FUNCTION_BLOCK "FB_CABINET_7P7-R22"
TITLE =Control cabinet 7P7-R22
{ S7_language := '9(1) Angielski (Stany Zjednoczone)  11.01.2022  09:45:15' }
VERSION : 0.1


VAR
  SM : STRUCT
   GeneralError : BOOL ;
   GeneralWarning : BOOL ;
   CtrlVoltageON : BOOL ;
   Auto : BOOL ;
   Manual : BOOL ;
   Local : BOOL ;
   Remote : BOOL ;
   CtrlRelease : BOOL ;
   CtrlRelease_A : BOOL ;
   res11 : BOOL ;
   res12 : BOOL ;
   res13 : BOOL ;
   res14 : BOOL ;
   res15 : BOOL ;
   LackCooling : BOOL ;
   LackHeating : BOOL ;
  END_STRUCT ;
  FM : STRUCT
   EnergyCounterFuse : BOOL ;
   ExternalVoltage400VAC : BOOL ;
   ControlVoltage24VDC : BOOL ;
   ControlVoltage230VAC_MS : BOOL ;
   CabinetCoolingFuse : BOOL ;
   ProfiNetSwitchFault : BOOL ;
   MainSwitchFault : BOOL ;
   ExcessTemperature : BOOL ;
   ESTOP : BOOL ;
   FireAlarmPreWarning : BOOL ;
   FireAlarm : BOOL ;
   MainSwitchEmgPower : BOOL ;
   NormElecBefMainSwitch : BOOL ;
   EmgElecBefMainSwitch : BOOL ;
   res16 : BOOL ;
   res17 : BOOL ;
  END_STRUCT ;
  CTRL : STRUCT
   ResetFault : BOOL ;
   ResetESTOP : BOOL ;
   LampTest : BOOL ;
   AutoStart : BOOL ;
   AutoStop : BOOL ;
   res05 : BOOL ;
   res06 : BOOL ;
   res07 : BOOL ;
   res10 : BOOL ;
   res11 : BOOL ;
   res12 : BOOL ;
   res13 : BOOL ;
   res14 : BOOL ;
   res15 : BOOL ;
   res16 : BOOL ;
   res17 : BOOL ;
  END_STRUCT ;
  CTRL_HMI : STRUCT
   ResetFault : BOOL ;
   Auto : BOOL ;
   Manual : BOOL ;
   res03 : BOOL ;
   res04 : BOOL ;
   res05 : BOOL ;
   res06 : BOOL ;
   res07 : BOOL ;
   ProductionOn : BOOL ;
   ProductionBreak : BOOL ;
   PlantOn : BOOL ;
   PlantOff : BOOL ;
   res14 : BOOL ;
   res15 : BOOL ;
   LackCooling : BOOL ;
   LackHeating : BOOL ;
  END_STRUCT ;
  EC : "UDT_EC";	//Energy Counter
END_VAR
VAR_TEMP
  ERROR_REL : BOOL ;
END_VAR
BEGIN
NETWORK
TITLE =STATUS



NETWORK
TITLE =CONTROL VOLTAGE ON
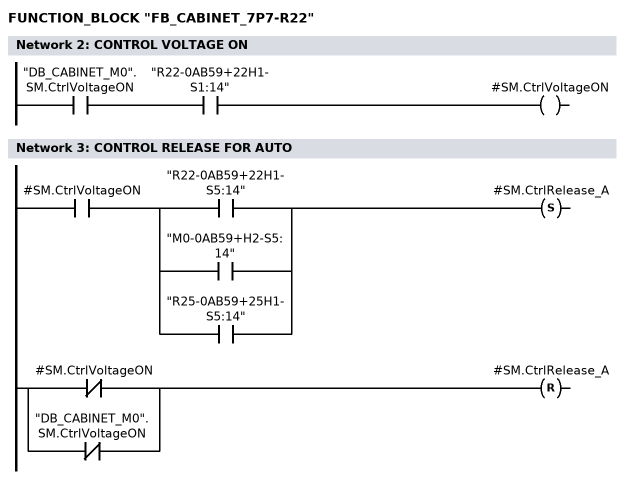
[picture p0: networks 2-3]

      U     "DB_CABINET_M0".SM.CtrlVoltageON;
      U     "R22-0AB59+22H1-S1:14";
      =     #SM.CtrlVoltageON;
NETWORK
TITLE =CONTROL RELEASE FOR AUTO

      U     #SM.CtrlVoltageON;
      U(    ;
      O     "R22-0AB59+22H1-S5:14";
      O     "M0-0AB59+H2-S5:14";
      O     "R25-0AB59+25H1-S5:14";
      )     ;
      S     #SM.CtrlRelease_A;
      U(    ;
      ON    #SM.CtrlVoltageON;
      ON    "DB_CABINET_M0".SM.CtrlVoltageON;
      )     ;
      R     #SM.CtrlRelease_A;
      NOP   0;
NETWORK
TITLE =AUTO/MANUAL MODE

      U(    ;
      U     "R22-0AB59+22H1-S2:14";
      S     #SM.Auto;
      U     "R22-0AB59+22H1-S2:22";
      R     #SM.Auto;
      U     #SM.Auto;
      )     ;
      NOT   ;
      =     #SM.Manual;
NETWORK
TITLE =LOCAL/REMOTE MODE

      U(    ;
      U     "DB_CABINET_M0".SM.Remote;
      S     #SM.Remote;
      U     "DB_CABINET_M0".SM.Local;
      R     #SM.Remote;
      U     #SM.Remote;
      )     ;
      NOT   ;
      =     #SM.Local;
NETWORK
TITLE =CONTROL RELEASE FROM CABINET
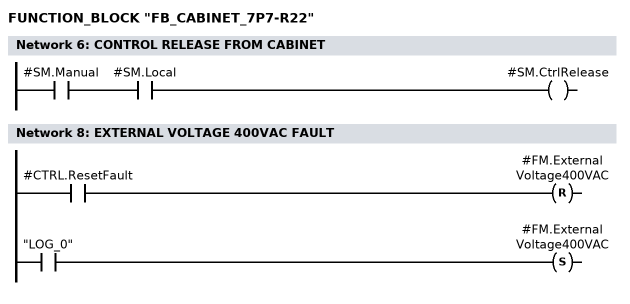
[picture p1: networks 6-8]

      U     #SM.Manual;
      U     #SM.Local;
      =     #SM.CtrlRelease;
NETWORK
TITLE =FAULTS



NETWORK
TITLE =EXTERNAL VOLTAGE 400VAC FAULT

      U     #CTRL.ResetFault;
      R     #FM.ExternalVoltage400VAC;
      U     "LOG_0";
      S     #FM.ExternalVoltage400VAC;
      NOP   0;
NETWORK
TITLE =CONTROL VOLTAGE 24V DC FAULT

      U     #CTRL.ResetFault;
      R     #FM.ControlVoltage24VDC;
      U(    ;
      O(    ;
      UN    "R22-0DC43+22H1-F1:7";
      L     S5T#300MS;
      SE    "T_R22-0DC43+22H1-F1";
      NOP   0;
      NOP   0;
      NOP   0;
      U     "T_R22-0DC43+22H1-F1";
      )     ;
      O(    ;
      UN    "R22-0DC43+22H1-F2:7";
      L     S5T#300MS;
      SE    "T_R22-0DC43+22H1-F2";
      NOP   0;
      NOP   0;
      NOP   0;
      U     "T_R22-0DC43+22H1-F2";
      )     ;
      )     ;
      S     #FM.ControlVoltage24VDC;
      NOP   0;
NETWORK
TITLE =CONTROL VOLTAGE 230VAC BEFORE MAIN SWITCH FAULT
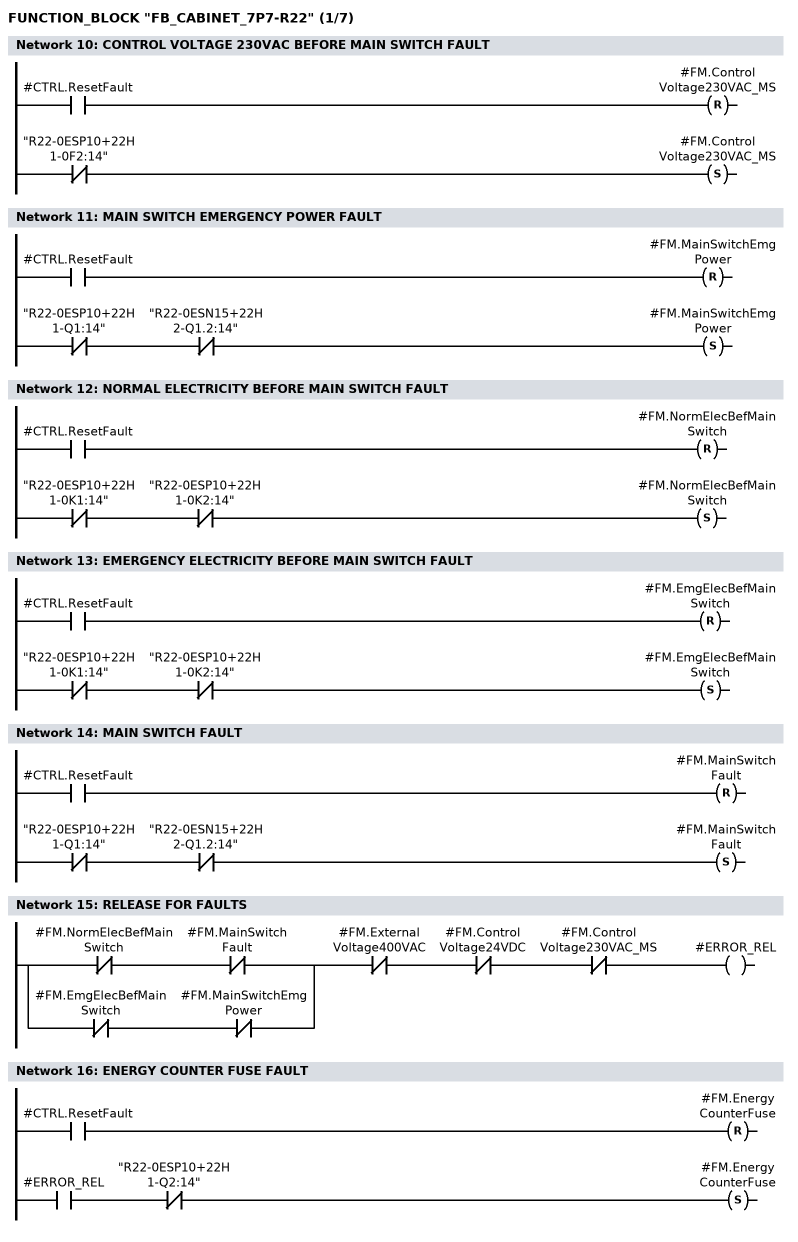
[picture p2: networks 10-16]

      U     #CTRL.ResetFault;
      R     #FM.ControlVoltage230VAC_MS;
      UN    "R22-0ESP10+22H1-0F2:14";
      S     #FM.ControlVoltage230VAC_MS;
      NOP   0;
NETWORK
TITLE =MAIN SWITCH EMERGENCY POWER FAULT

      U     #CTRL.ResetFault;
      R     #FM.MainSwitchEmgPower;
      UN    "R22-0ESP10+22H1-Q1:14";
      UN    "R22-0ESN15+22H2-Q1.2:14";
      S     #FM.MainSwitchEmgPower;
      NOP   0;
NETWORK
TITLE =NORMAL ELECTRICITY BEFORE MAIN SWITCH FAULT

      U     #CTRL.ResetFault;
      R     #FM.NormElecBefMainSwitch;
      UN    "R22-0ESP10+22H1-0K1:14";
      UN    "R22-0ESP10+22H1-0K2:14";
      S     #FM.NormElecBefMainSwitch;
      NOP   0;
NETWORK
TITLE =EMERGENCY ELECTRICITY BEFORE MAIN SWITCH FAULT

      U     #CTRL.ResetFault;
      R     #FM.EmgElecBefMainSwitch;
      UN    "R22-0ESP10+22H1-0K1:14";
      UN    "R22-0ESP10+22H1-0K2:14";
      S     #FM.EmgElecBefMainSwitch;
      NOP   0;
NETWORK
TITLE =MAIN SWITCH FAULT

      U     #CTRL.ResetFault;
      R     #FM.MainSwitchFault;
      UN    "R22-0ESP10+22H1-Q1:14";
      UN    "R22-0ESN15+22H2-Q1.2:14";
      S     #FM.MainSwitchFault;
      NOP   0;
NETWORK
TITLE =RELEASE FOR FAULTS

      U(    ;
      UN    #FM.NormElecBefMainSwitch;
      UN    #FM.MainSwitchFault;
      O     ;
      UN    #FM.EmgElecBefMainSwitch;
      UN    #FM.MainSwitchEmgPower;
      )     ;
      UN    #FM.ExternalVoltage400VAC;
      UN    #FM.ControlVoltage24VDC;
      UN    #FM.ControlVoltage230VAC_MS;
      =     #ERROR_REL;
NETWORK
TITLE =ENERGY COUNTER FUSE FAULT

      U     #CTRL.ResetFault;
      R     #FM.EnergyCounterFuse;
      U     #ERROR_REL;
      UN    "R22-0ESP10+22H1-Q2:14";
      S     #FM.EnergyCounterFuse;
      NOP   0;
NETWORK
TITLE =CABINET COOLING FUSE FAULT
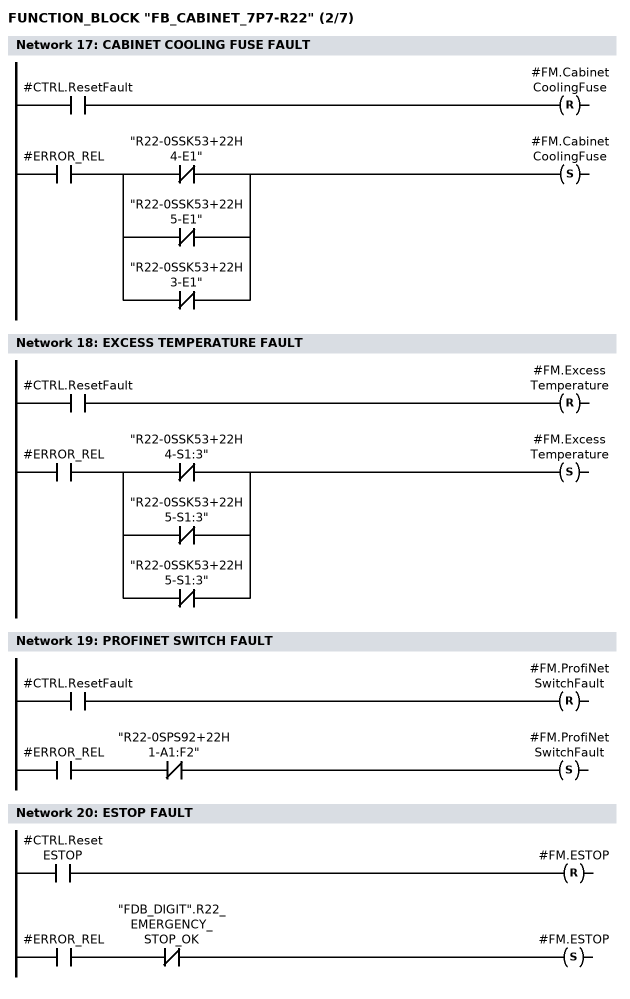
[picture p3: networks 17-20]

      U     #CTRL.ResetFault;
      R     #FM.CabinetCoolingFuse;
      U     #ERROR_REL;
      U(    ;
      ON    "R22-0SSK53+22H4-E1";
      ON    "R22-0SSK53+22H5-E1";
      ON    "R22-0SSK53+22H3-E1";
      )     ;
      S     #FM.CabinetCoolingFuse;
      NOP   0;
NETWORK
TITLE =EXCESS TEMPERATURE FAULT

      U     #CTRL.ResetFault;
      R     #FM.ExcessTemperature;
      U     #ERROR_REL;
      U(    ;
      ON    "R22-0SSK53+22H4-S1:3";
      ON    "R22-0SSK53+22H5-S1:3";
      ON    "R22-0SSK53+22H5-S1:3";
      )     ;
      S     #FM.ExcessTemperature;
      NOP   0;
NETWORK
TITLE =PROFINET SWITCH FAULT

      U     #CTRL.ResetFault;
      R     #FM.ProfiNetSwitchFault;
      U     #ERROR_REL;
      UN    "R22-0SPS92+22H1-A1:F2";
      S     #FM.ProfiNetSwitchFault;
      NOP   0;
NETWORK
TITLE =ESTOP FAULT

      U     #CTRL.ResetESTOP;
      R     #FM.ESTOP;
      U     #ERROR_REL;
      UN    "FDB_DIGIT".R22_EMERGENCY_STOP_OK;
      S     #FM.ESTOP;
      NOP   0;
NETWORK
TITLE =GENERAL FAULT / WARNING
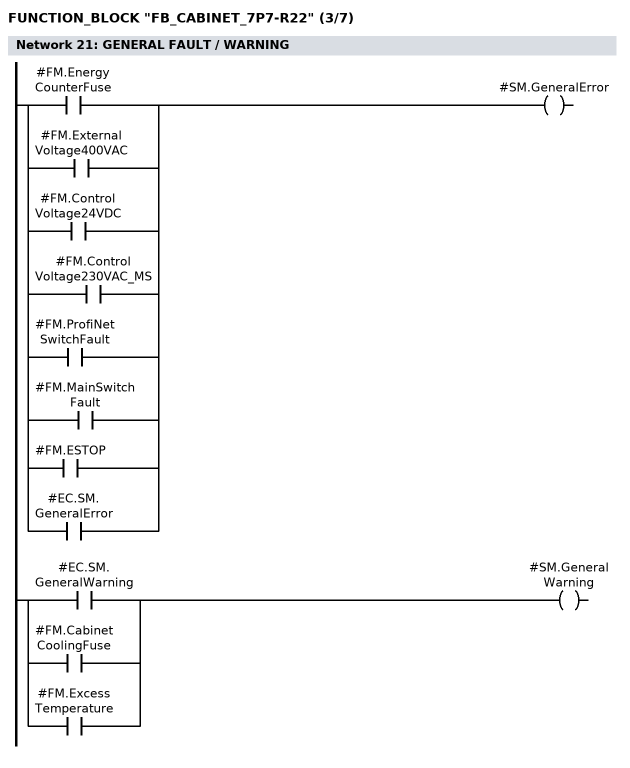
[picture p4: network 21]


      U     #FM.EnergyCounterFuse;
      O     #FM.ExternalVoltage400VAC;
      O     #FM.ControlVoltage24VDC;
      O     #FM.ControlVoltage230VAC_MS;
      O     #FM.ProfiNetSwitchFault;
      O     #FM.MainSwitchFault;
      O     #FM.ESTOP;
      O     #EC.SM.GeneralError;
      =     #SM.GeneralError;


      U     #EC.SM.GeneralWarning;
      O     #FM.CabinetCoolingFuse;
      O     #FM.ExcessTemperature;
      =     #SM.GeneralWarning;

NETWORK
TITLE =CONTROL SIGNALS



NETWORK
TITLE =RESET FAULT
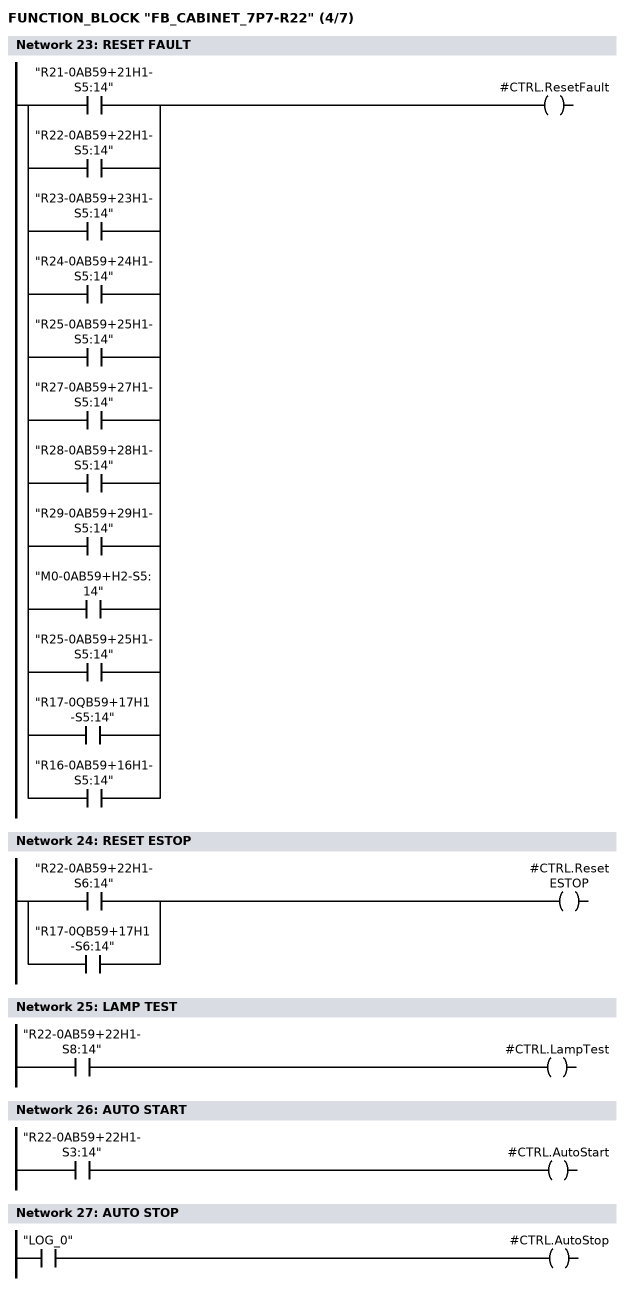
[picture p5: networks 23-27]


      O     "R21-0AB59+21H1-S5:14";
      O     "R22-0AB59+22H1-S5:14";
      O     "R23-0AB59+23H1-S5:14";
      O     "R24-0AB59+24H1-S5:14";
      O     "R25-0AB59+25H1-S5:14";
      O     "R27-0AB59+27H1-S5:14";
      O     "R28-0AB59+28H1-S5:14";
      O     "R29-0AB59+29H1-S5:14";
      O     "M0-0AB59+H2-S5:14";
      O     "R25-0AB59+25H1-S5:14";
      O     "R17-0QB59+17H1-S5:14";
      O     "R16-0AB59+16H1-S5:14";
      =     #CTRL.ResetFault;
NETWORK
TITLE =RESET ESTOP



      O     "R22-0AB59+22H1-S6:14";
      O     "R17-0QB59+17H1-S6:14";
      =     #CTRL.ResetESTOP;
NETWORK
TITLE =LAMP TEST



      U     "R22-0AB59+22H1-S8:14";
      =     #CTRL.LampTest;
NETWORK
TITLE =AUTO START



      U     "R22-0AB59+22H1-S3:14";
      =     #CTRL.AutoStart;
NETWORK
TITLE =AUTO STOP



      U     "LOG_0";
      =     #CTRL.AutoStop;
NETWORK
TITLE =BUTTON LAMPS
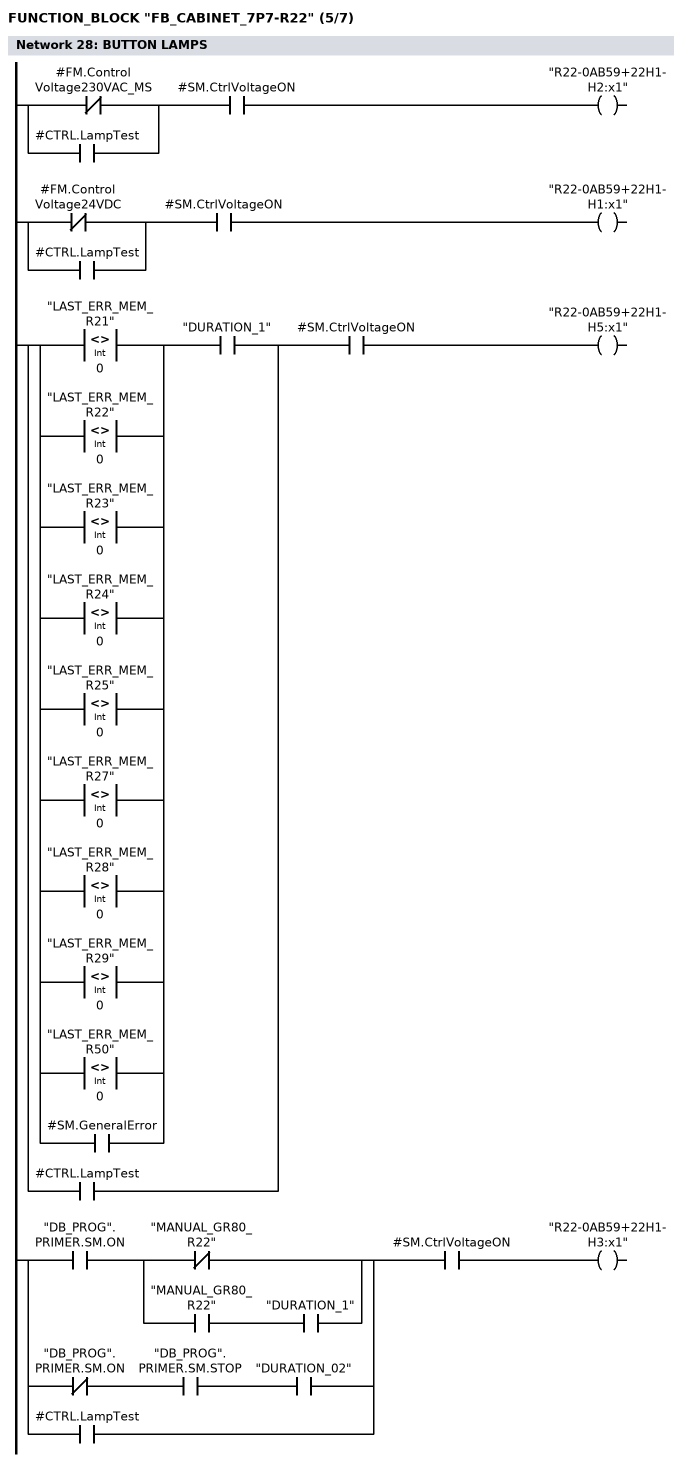
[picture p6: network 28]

// CONTROL VOLTAGE 230V AC
      U(    ;
      ON    #FM.ControlVoltage230VAC_MS;
      O     #CTRL.LampTest;
      )     ;
      U     #SM.CtrlVoltageON;
      =     "R22-0AB59+22H1-H2:x1";

// CONTROL VOLTAGE 24V DC
      U(    ;
      ON    #FM.ControlVoltage24VDC;
      O     #CTRL.LampTest;
      )     ;
      U     #SM.CtrlVoltageON;
      =     "R22-0AB59+22H1-H1:x1";

// RESET
      U(    ;
      L     "LAST_ERR_MEM_R21";
      L     0;
      <>I   ;
      )     ;
      O(    ;
      L     "LAST_ERR_MEM_R22";
      L     0;
      <>I   ;
      )     ;
      O(    ;
      L     "LAST_ERR_MEM_R23";
      L     0;
      <>I   ;
      )     ;
      O(    ;
      L     "LAST_ERR_MEM_R24";
      L     0;
      <>I   ;
      )     ;
      O(    ;
      L     "LAST_ERR_MEM_R25";
      L     0;
      <>I   ;
      )     ;
      O(    ;
      L     "LAST_ERR_MEM_R27";
      L     0;
      <>I   ;
      )     ;
      O(    ;
      L     "LAST_ERR_MEM_R28";
      L     0;
      <>I   ;
      )     ;
      O(    ;
      L     "LAST_ERR_MEM_R29";
      L     0;
      <>I   ;
      )     ;
      O(    ;
      L     "LAST_ERR_MEM_R50";
      L     0;
      <>I   ;
      )     ;
      O     #SM.GeneralError;
      U     "DURATION_1";
      O     #CTRL.LampTest;
      U     #SM.CtrlVoltageON;
      =     "R22-0AB59+22H1-H5:x1";

// AUTOMATIC START
      U(    ;
      U     "DB_PROG".PRIMER.SM.ON;
      U(    ;
      ON    "MANUAL_GR80_R22";
      O     ;
      U     "MANUAL_GR80_R22";
      U     "DURATION_1";
      )     ;
      O     ;
      UN    "DB_PROG".PRIMER.SM.ON;
      U     "DB_PROG".PRIMER.SM.STOP;
      U     "DURATION_02";
      O     #CTRL.LampTest;
      )     ;
      U     #SM.CtrlVoltageON;
      =     "R22-0AB59+22H1-H3:x1";
NETWORK
TITLE =LIGHT TOWER
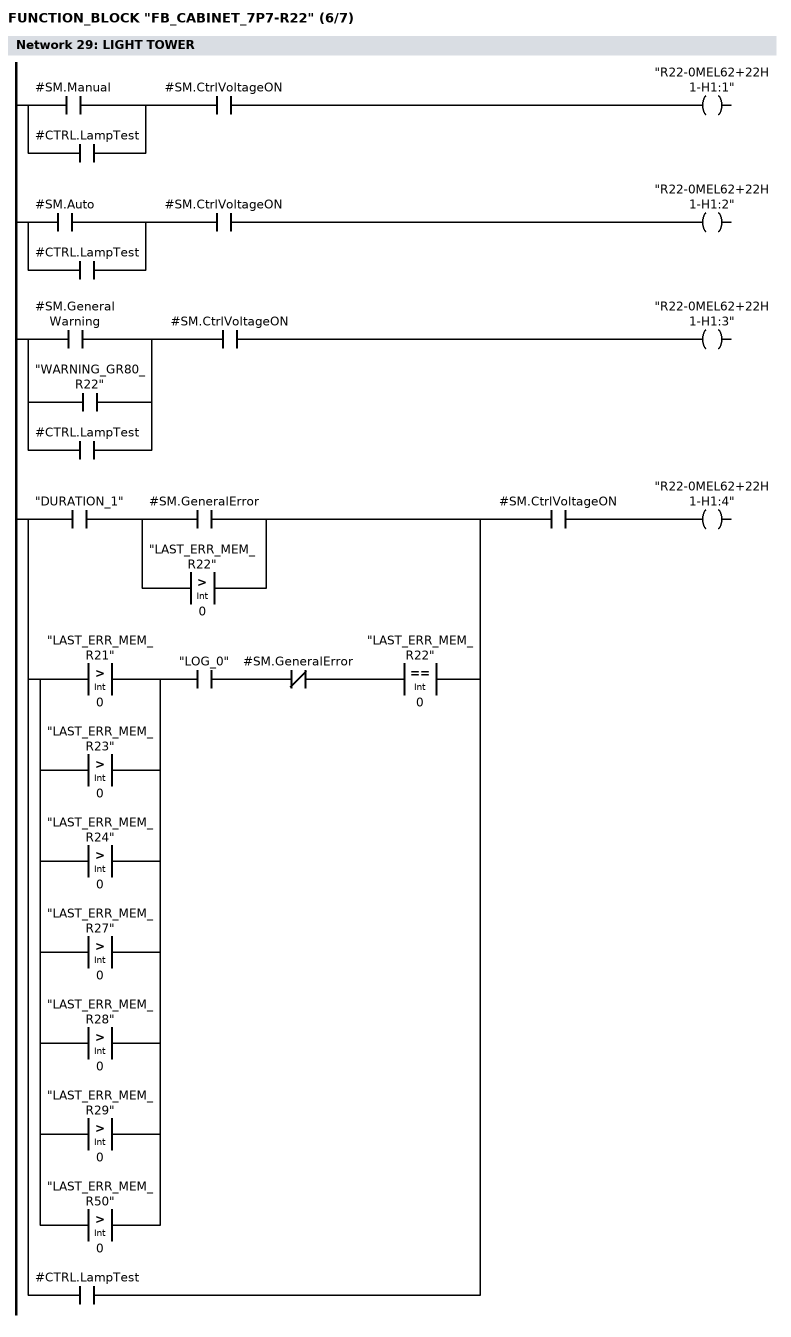
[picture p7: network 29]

// MANUAL
      U(    ;
      O     #SM.Manual;
      O     #CTRL.LampTest;
      )     ;
      U     #SM.CtrlVoltageON;
      =     "R22-0MEL62+22H1-H1:1";

// AUTO
      U(    ;
      O     #SM.Auto;
      O     #CTRL.LampTest;
      )     ;
      U     #SM.CtrlVoltageON;
      =     "R22-0MEL62+22H1-H1:2";

// WARNING
      U(    ;
      O     #SM.GeneralWarning;
      O     "WARNING_GR80_R22";
      O     #CTRL.LampTest;
      )     ;
      U     #SM.CtrlVoltageON;
      =     "R22-0MEL62+22H1-H1:3";

// FAULT
      U(    ;
      U     "DURATION_1";
      U(    ;
      O     #SM.GeneralError;
      O(    ;
      L     "LAST_ERR_MEM_R22";
      L     0;
      >I    ;
      )     ;
      )     ;
      O     ;
      U(    ;
      O(    ;
      L     "LAST_ERR_MEM_R21";
      L     0;
      >I    ;
      )     ;
      O(    ;
      L     "LAST_ERR_MEM_R23";
      L     0;
      >I    ;
      )     ;
      O(    ;
      L     "LAST_ERR_MEM_R24";
      L     0;
      >I    ;
      )     ;
      O(    ;
      L     "LAST_ERR_MEM_R27";
      L     0;
      >I    ;
      )     ;
      O(    ;
      L     "LAST_ERR_MEM_R28";
      L     0;
      >I    ;
      )     ;
      O(    ;
      L     "LAST_ERR_MEM_R29";
      L     0;
      >I    ;
      )     ;
      O(    ;
      L     "LAST_ERR_MEM_R50";
      L     0;
      >I    ;
      )     ;
      )     ;
      U     "LOG_0";
      UN    #SM.GeneralError;
      U(    ;
      L     "LAST_ERR_MEM_R22";
      L     0;
      ==I   ;
      )     ;
      O     #CTRL.LampTest;
      )     ;
      U     #SM.CtrlVoltageON;
      =     "R22-0MEL62+22H1-H1:4";
NETWORK
TITLE =HORN
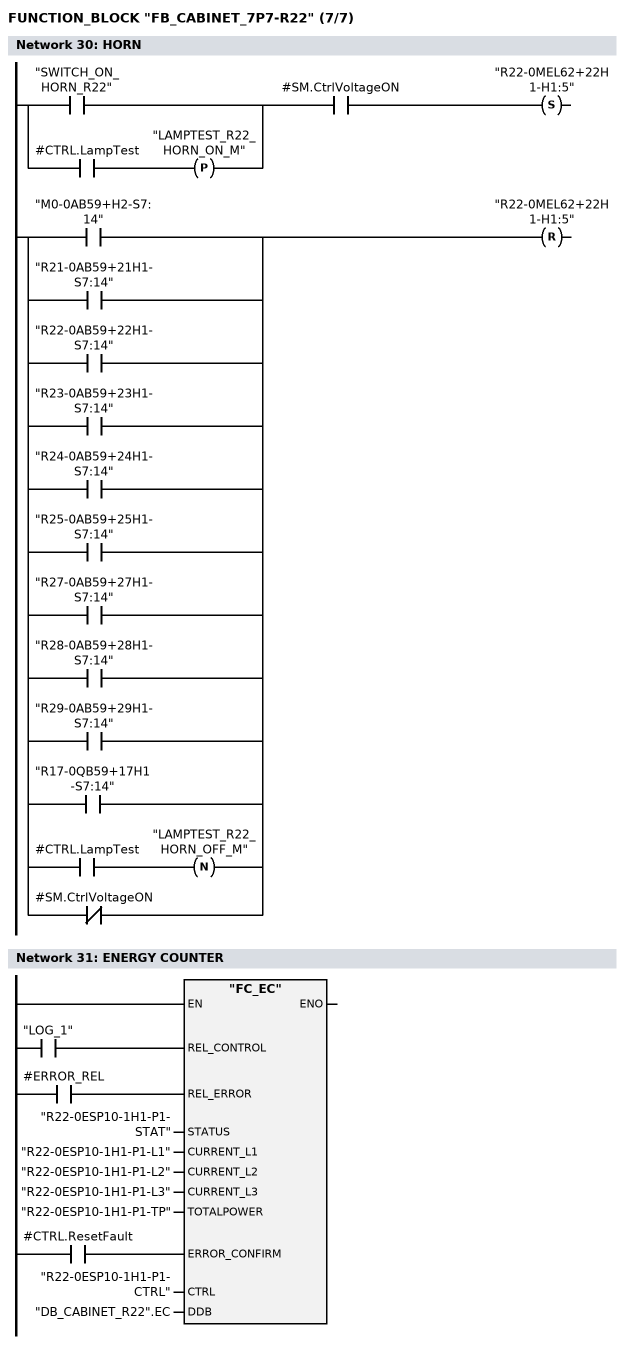
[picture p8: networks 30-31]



      U(    ;
      O     "SWITCH_ON_HORN_R22";
      O(    ;
      U     #CTRL.LampTest;
      FP    "LAMPTEST_R22_HORN_ON_M";
      )     ;
      )     ;
      U     #SM.CtrlVoltageON;
      S     "R22-0MEL62+22H1-H1:5";
      U(    ;
      O     "M0-0AB59+H2-S7:14";
      O     "R21-0AB59+21H1-S7:14";
      O     "R22-0AB59+22H1-S7:14";
      O     "R23-0AB59+23H1-S7:14";
      O     "R24-0AB59+24H1-S7:14";
      O     "R25-0AB59+25H1-S7:14";
      O     "R27-0AB59+27H1-S7:14";
      O     "R28-0AB59+28H1-S7:14";
      O     "R29-0AB59+29H1-S7:14";
      O     "R17-0QB59+17H1-S7:14";
      O(    ;
      U     #CTRL.LampTest;
      FN    "LAMPTEST_R22_HORN_OFF_M";
      )     ;
      ON    #SM.CtrlVoltageON;
      )     ;
      R     "R22-0MEL62+22H1-H1:5";
      NOP   0;
NETWORK
TITLE =ENERGY COUNTER

      U     "LOG_1";
      =     L      1.0;
      BLD   103;
      U     #ERROR_REL;
      =     L      1.1;
      BLD   103;
      U     #CTRL.ResetFault;
      =     L      1.2;
      BLD   103;
      CALL "FC_EC" (
           REL_CONTROL              := L      1.0,
           REL_ERROR                := L      1.1,
           STATUS                   := "R22-0ESP10-1H1-P1-STAT",
           CURRENT_L1               := "R22-0ESP10-1H1-P1-L1",
           CURRENT_L2               := "R22-0ESP10-1H1-P1-L2",
           CURRENT_L3               := "R22-0ESP10-1H1-P1-L3",
           TOTALPOWER               := "R22-0ESP10-1H1-P1-TP",
           ERROR_CONFIRM            := L      1.2,
           CTRL                     := "R22-0ESP10-1H1-P1-CTRL",
           DDB                      := "DB_CABINET_R22".EC);
      NOP   0;
NETWORK
TITLE =END



END_FUNCTION_BLOCK

